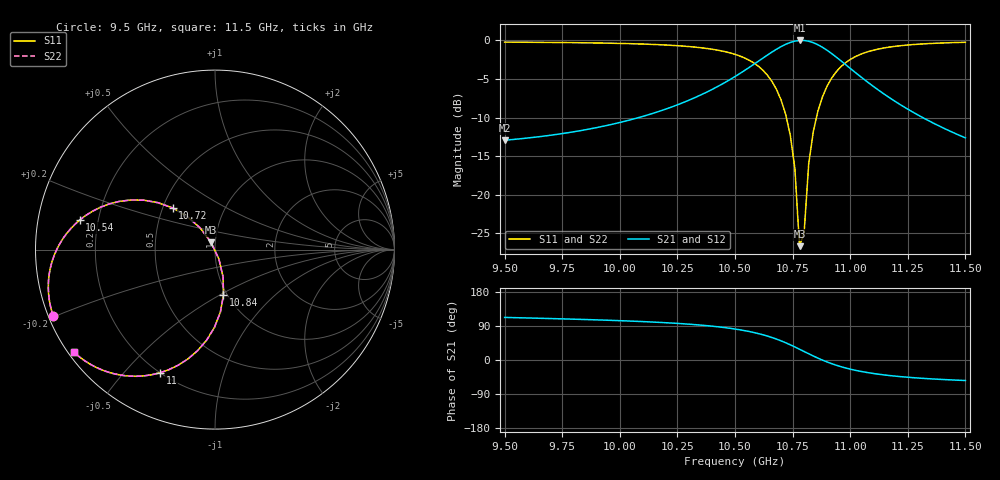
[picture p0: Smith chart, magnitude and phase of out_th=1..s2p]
!freq-unit param-type data-format keyword impedance-ohms
# GHZ  S  MA  R  50
!Freq  MagS11 AngS11 MagS21  AngS21 MagS12 AngS12
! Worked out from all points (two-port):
!   101 points, 9.5 GHz to 11.5 GHz, reference 50 ohm
!   highest |S21| = -0.01 dB at 10.78 GHz (marker M1); lowest = -12.9 dB at 9.5 GHz (marker M2)
!   |S21| within 3 dB of the highest: 10.59 GHz to 10.97 GHz (388.8 MHz wide, 3.61 % of centre)
!   lowest |S11| = -26.6 dB at 10.78 GHz (marker M3), VSWR 1.10, Z = 47.7 + j3.91 ohm
!   |S11| at or under -10 dB: 10.72 GHz to 10.85 GHz (130.4 MHz wide, 1.21 % of centre)
!   |S22| runs from -26.6 to -0.2 dB; largest |S21 - S12| = 0
!   S11 on the Smith chart (normalised r, x): 9.5 GHz: 0.01, -0.20; 10.54 GHz: 0.13, +0.11; 10.72 GHz: 0.56, +0.29; 10.84 GHz: 0.96, -0.52; 11 GHz: 0.20, -0.63; 11.5 GHz: 0.02, -0.32
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9.5  0.9742 -157.6  0.2259 112.4  0.2259 112.4  0.9742 -157.6
9.84  0.965 -163.0  0.2622 107.0  0.2622 107.0  0.965 -163.0
10.18  0.9364 -171.0  0.351 99.0  0.351 99.0  0.9364 -171.0
10.38  0.8855 -179.5  0.4647 90.5  0.4647 90.5  0.8855 -179.5
10.5  0.8122 171.7  0.5834 81.7  0.5834 81.7  0.8122 171.7
10.54  0.7715 167.7  0.6363 77.7  0.6363 77.7  0.7715 167.7
10.64  0.5971 153.3  0.8022 63.3  0.8022 63.3  0.5971 153.3
10.68  0.4818 145.2  0.8763 55.2  0.8763 55.2  0.4818 145.2
10.72  0.3316 135.5  0.9434 45.5  0.9434 45.5  0.3316 135.5
10.74  0.2432 130.1  0.97 40.1  0.97 40.1  0.2432 130.1
10.76  0.1475 124.4  0.9891 34.4  0.9891 34.4  0.1475 124.4
10.78  0.04655 118.5  0.9989 28.5  0.9989 28.5  0.04655 118.5
10.8  0.0568 -67.6  0.9984 22.4  0.9984 22.4  0.0568 -67.6
10.82  0.1592 -73.6  0.9872 16.4  0.9872 16.4  0.1592 -73.6
10.84  0.2576 -79.4  0.9662 10.6  0.9662 10.6  0.2576 -79.4
10.86  0.3493 -85.1  0.937 4.9  0.937 4.9  0.3493 -85.1
10.9  0.5068 -95.3  0.8621 -5.3  0.8621 -5.3  0.5068 -95.3
10.94  0.6277 -103.9  0.7785 -13.9  0.7785 -13.9  0.6277 -103.9
11  0.7518 -114.1  0.6594 -24.1  0.6594 -24.1  0.7518 -114.1
11.08  0.8474 -123.7  0.5309 -33.7  0.5309 -33.7  0.8474 -123.7
11.18  0.9091 -131.6  0.4166 -41.6  0.4166 -41.6  0.9091 -131.6
11.5  0.9723 -144.1  0.2339 -54.1  0.2339 -54.1  0.9723 -144.1
